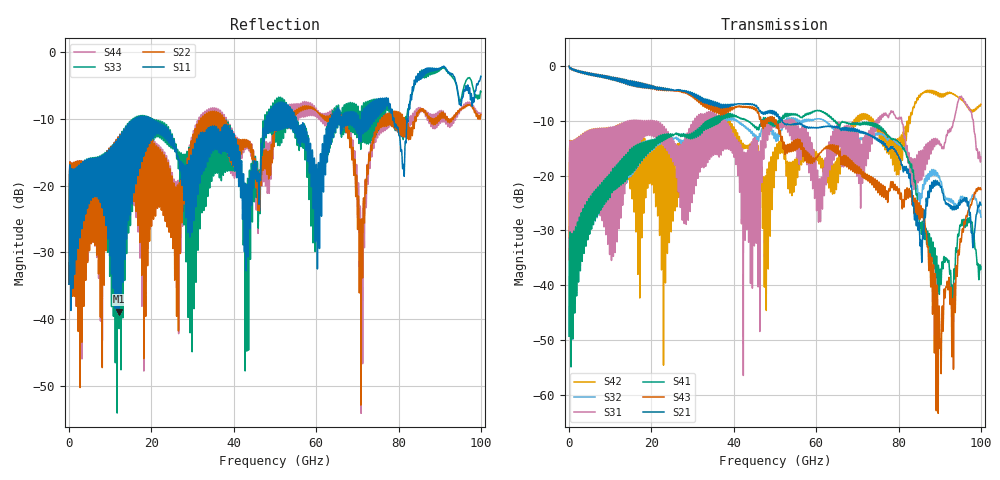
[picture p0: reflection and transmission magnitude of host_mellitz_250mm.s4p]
# Hz S RI R 50
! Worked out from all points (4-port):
!   10000 points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, 10 MHz to 100 GHz, reference 50 ohm
!   strongest paths, dB at 10 MHz, 25.01 GHz, 50.01 GHz, 75.01 GHz, 100 GHz:
!     S21: -0.1, -4.4, -8.9, -13.6, -25.4
!     S43: -0.1, -4.6, -10.6, -23.1, -22.5
!     S41: -49.3, -12.5, -10.4, -11.0, -36.6
!     S31: -35.3, -13.8, -10.7, -10.0, -16.6
!     S32: -49.3, -13.1, -12.4, -12.2, -27.6
!     S42: -35.3, -14.4, -15.0, -11.9, -7.0
!   lowest |S11| = -38.9 dB at 12.12 GHz (marker M1), VSWR 1.02, Z = 51.1 + j0.11 ohm
!   |S11| at or under -10 dB: start of sweep to 16 GHz; 19.79 GHz to 48.02 GHz (28.23 GHz wide, 83.2 % of centre); 55.04 GHz to 63.38 GHz (8.338 GHz wide, 14.1 % of centre)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
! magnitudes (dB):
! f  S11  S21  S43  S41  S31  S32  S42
! 10 MHz  -34.8  -0.1  -0.1  -49.3  -35.3  -49.3  -35.3
! 12.12 GHz  -38.9  -2.3  -2.3  -20.3  -26.9  -20.8  -19.0
! 65.65 GHz  -8.9  -11.5  -15.9  -11.1  -13.3  -12.4  -16.3
! 70.88 GHz  -13.4  -11.9  -19.0  -10.4  -18.4  -13.1  -9.9
! 74.02 GHz  -10.2  -12.9  -22.1  -10.4  -12.7  -12.5  -11.2
! 90.03 GHz  -2.4  -21.8  -50.2  -38.0  -14.3  -20.6  -5.3
! 100 GHz  -3.6  -25.4  -22.5  -36.6  -16.6  -27.6  -7.0
